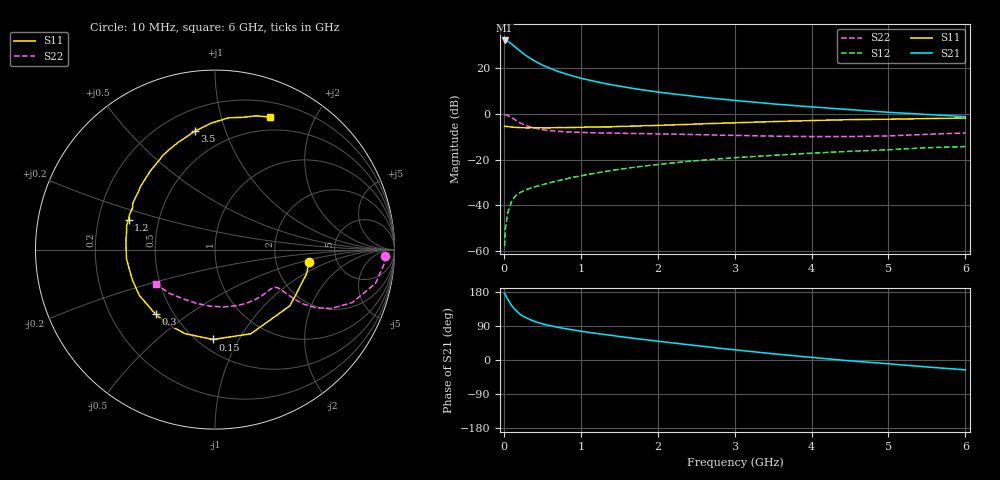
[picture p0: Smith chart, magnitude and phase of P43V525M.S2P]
! SIEMENS Small Signal Semiconductors
! BFP182
! Si NPN RF Bipolar Junction Transistor in SOT143
! VCE = 3.5 V  IC = 25 mA
! Common Emitter S-Parameters:  March  1996
# GHz  S  MA  R  50
!  f  S11  S21  S12  S22
! GHz  MAG  ANG  MAG  ANG  MAG  ANG  MAG  ANG
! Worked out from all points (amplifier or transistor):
!   36 points, 10 MHz to 6 GHz, reference 50 ohm
!   highest |S21| = 31.8 dB at 10 MHz (marker M1)
!   |S21| within 3 dB of that: start of sweep to 153.7 MHz
!   unconditionally stable (mu >= 1): 635.7 MHz to 5.394 GHz
!   at 250 MHz: K = 0.58, MSG = 30.0 dB, |S12| = -33.8 dB
!   at 1.4 GHz: K = 1.21, MAG = 15.9 dB, |S12| = -24.8 dB
!   at 6 GHz: K = 0.94, MSG = 6.5 dB, |S12| = -14.3 dB
!   S11 on the Smith chart (normalised r, x): 10 MHz: 3.12, -0.60; 150 MHz: 0.59, -0.78; 300 MHz: 0.40, -0.38; 1.2 GHz: 0.33, +0.15; 3.5 GHz: 0.33, +0.79; 6 GHz: 0.35, +1.44
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0.01  0.5288 -7.5  39.08 175.8  0.0013 83.1  0.9478 -2.1
0.02  0.5277 -15.0  39.03 172.3  0.0031 75.3  0.9471 -4.7
0.05  0.5219 -36.8  37.65 160.6  0.0068 78.7  0.9138 -11.9
0.1  0.5097 -67.0  32.77 144.4  0.0121 63.9  0.8198 -21.1
0.15  0.5009 -91.5  27.99 131.9  0.0162 58.2  0.7258 -26.9
0.2  0.4971 -109.8  23.85 122.5  0.0186 54.7  0.6467 -30.0
0.25  0.4926 -122.9  20.43 115.6  0.0205 51.9  0.5854 -31.5
0.3  0.489 -132.6  17.8 110.3  0.0224 51.2  0.5416 -31.9
0.4  0.4928 -148.6  13.97 101.6  0.0255 52.1  0.4816 -31.8
0.5  0.4904 -159.7  11.39 95.5  0.0282 51.8  0.4471 -31.5
0.6  0.4898 -167.3  9.696 90.6  0.0312 53.6  0.4262 -31.3
0.7  0.4963 -174.5  8.304 86.4  0.0345 54.8  0.4118 -31.3
0.8  0.4951 179.2  7.358 82.7  0.0375 54.9  0.4019 -31.7
1.1  0.5099 164.8  5.397 73.0  0.0477 56.0  0.3848 -34.0
1.2  0.5097 160.9  4.949 70.4  0.0509 56.1  0.381 -35.1
1.7  0.5339 143.2  3.479 57.0  0.0682 54.6  0.3685 -42.3
2.2  0.568 129.3  2.679 44.9  0.0845 51.0  0.3576 -51.3
2.8  0.615 113.9  2.086 31.1  0.1034 46.0  0.3398 -64.0
3.5  0.6695 99.7  1.626 16.5  0.1234 39.7  0.3228 -81.5
4.5  0.7383 84.1  1.219 -2.2  0.1509 31.1  0.3167 -109.5
5.5  0.7793 73.0  0.958 -18.4  0.1805 22.8  0.3538 -136.9
6  0.7994 67.5  0.856 -26.0  0.192 17.6  0.379 -149.8
